FUNCTION_BLOCK FB_DO_IED_LD1_MMXU1_TotW EXTENDS FB_AcsiCommonDataClass
VAR_INPUT
	mag: FB_AcsiDATypeAnalogueValue := (fc:=ACSI_FC_MX, TrgOp:=ACSI_TrgOp_dchg OR ACSI_TrgOp_dupd, bLinkResult:=THIS^.AddDataToContainer(ipData:=mag));
	q: FB_AcsiDATypeQuality := (fc:=ACSI_FC_MX, TrgOp:=ACSI_TrgOp_qchg, bLinkResult:=THIS^.AddDataToContainer(ipData:=q));
	t: FB_AcsiDATypeTimeStamp := (fc:=ACSI_FC_MX, bLinkResult:=THIS^.AddDataToContainer(ipData:=t));
	units: FB_AcsiDATypeUnit := (fc:=ACSI_FC_CF, TrgOp:=ACSI_TrgOp_dchg, SIUnit:=(eValue:=E_AcsiSIUnit.Watt), multiplier:=(eValue:=E_AcsiMultiplier.Kilo, bPresence:=TRUE), bLinkResult:=THIS^.AddDataToContainer(ipData:=units));
END_VAR
VAR
END_VAR

(* User application data update event method. *)
METHOD OnGetVPreEvent : E_AcsiServiceError
VAR_INPUT
	ipDai : I_AcsiDataAccessInfoClass;(* Additional data access info *)
	ipData : I_AcsiCommonDataClass;(* Interface pointer to data object *)
	eFc	: E_AcsiFc;(* Functional constraint *)
END_VAR
VAR
	ipAssociation : I_ScsmAssociationClass;
	tT : T_UtcTime;
END_VAR
(* This implementation is only for demonstration purposes. *)

(* ScsmAssociation_From_Dai() function queries the ipDai for SCSM association interface pointer information. *)
IF ScsmAssociation_From_Dai(in:=ipDai, out=>ipAssociation) THEN

	(* Check if attribute 'f' value is read by remote communication partner. *)
	IF ipData.sObjectName = 'f' THEN
		
		(* Modify/simulate new attribute 'f' (analogue value) or get the value from analogue input terminal or some other sensor. *)
		mag.f.fValue:=SEL(mag.f.fValue < 100.0, 0, mag.f.fValue + 10.1);

		(* Modify/simulate attribute 'q' (quality). *)
		q.eValidity:=SEL(q.eValidity = E_AcsiQualityValidity.Good, SEL(q.eValidity = E_AcsiQualityValidity.Invalid, E_AcsiQualityValidity.Good, E_AcsiQualityValidity.Questionable), E_AcsiQualityValidity.Invalid);
		q.eSource:=SEL(q.eSource = E_AcsiQualitySource.Process, E_AcsiQualitySource.Process, E_AcsiQualitySource.Substituted);
		q.Test:=NOT q.Test;
		q.OutOfRange:=SEL(mag.f.fValue > 50.0, FALSE, TRUE);

		(* Use of the SCSM association interface to get new time-stamp value. *)
		IF ipAssociation.GetSystemTime(tT=>tT) THEN
			t.tValue:=tT;(* Set/refresh the 't' attribute value (time-stamp). *)
		END_IF
	END_IF
END_IF

//OnGetVPreEvent:=E_AcsiServiceError.NoError; (* Default return value => not mandatory *)
END_METHOD

END_FUNCTION_BLOCK
